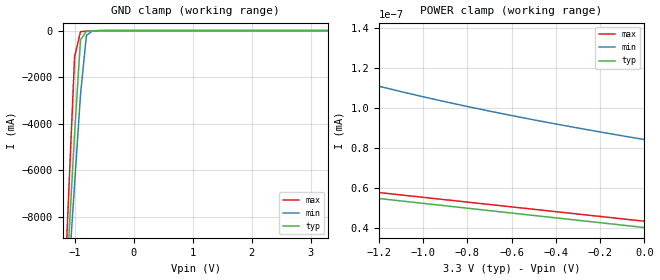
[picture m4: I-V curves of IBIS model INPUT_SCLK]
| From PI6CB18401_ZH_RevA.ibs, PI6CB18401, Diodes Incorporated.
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|   Model INPUT_SCLK
[Model] INPUT_SCLK
Model_type Input
Vinl = 990.00mV
Vinh = 2.3100V
| variable   typ   min   max
C_comp   1.000pF   0.997pF   2.003pF
[Voltage Range]   3.3000V   3.0000V   3.6000V
[POWER Clamp Reference]   3.3000V   3.0000V   3.6000V
[GND Clamp Reference]   0.0000V   0.0000V   0.0000V
[Temperature Range]   25   85   -40
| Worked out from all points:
|   GND clamp passes 1 mA (typ) near -0.52 V on its own axis
|   POWER clamp passes 1 mA (typ) near -2.41 V on its own axis
[GND Clamp]
| Voltage   I(typ)   I(min)   I(max)
-3.3V     -110.4A    -94.87A    -136.7A
-1.2V     -13.62A    -14.27A    -12.9A
-1.1V     -9.015A    -10.43A    -7.011A
-1V       -4.408A    -6.598A    -1.127A
-900mV    -398.5mA   -2.763A    -46.09mA
-800mV    -34.09mA   -202.3mA   -27.12mA
-700mV    -13.65mA   -21.62mA   -12.43mA
3.3V      40.05pA    89.93pA    39.6pA
[POWER Clamp]
| Voltage   I(typ)   I(min)   I(max)
-3.3V     31.96A     18.04A     54A
-2.1V     1.794nA    176.3pA    444.5nA
-2V       101.8pA    138.5pA    3.374nA
-1.9V     63.98pA    133.4pA    90.6pA
-1.8V     61.96pA    129.7pA    64.98pA
-1.4V     57.04pA    116.6pA    60pA
-1V       52.17pA    105.6pA    55.2pA
-500mV    46.1pA     94.04pA    49.2pA
0V        40.05pA    84.16pA    43.2pA
